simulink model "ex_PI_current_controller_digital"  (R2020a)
settings: Solver=ode45  StartTime=0.0  StopTime=0.1  MaxStep=1e-6  RelTol=1e-4  AbsTol=1e-6  EnableMultiTasking=on
libraries: powerlib x4

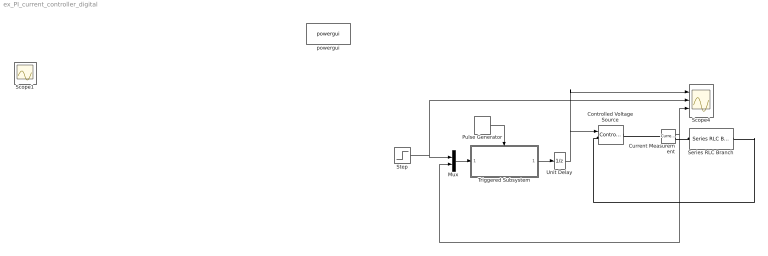
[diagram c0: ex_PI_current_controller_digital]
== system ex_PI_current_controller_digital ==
  Controlled Voltage Source : powerlib/Electrical Sources/Controlled Voltage Source  Initialize=on  Source_Type=AC  Amplitude=0  Phase=0  Frequency=0  Measurements=None
  Current Measurement : powerlib/Measurements/Current Measurement  PhasorSimulation=off  OutputType=Complex  PSBequivalent=0
  Mux : Mux  Inputs=2
  Pulse Generator : DiscretePulseGenerator  PulseType=Time based  Period=0.0001  PulseWidth=50
  Scope4 : Scope  NumInputPorts=3
  Series RLC Branch : powerlib/Elements/Series RLC Branch  LConnTagsString=__new0  RConnTagsString=__new0  BranchType=RL  Resistance=0.1  Inductance=0.001  SetiL0=off  InitialCurrent=0  Capacitance=1e-6  Setx0=off  InitialVoltage=0  Measurements=None
  Step : Step  Time=0.02  After=10  SampleTime=0
  Triggered Subsystem : Subsystem  TreatAsAtomicUnit=on
  Unit Delay : UnitDelay  SampleTime=0.0001  HasFrameUpgradeWarning=on
  powergui : powerlib/powergui  Priority=1  SimulationMode=Continuous  SampleTime=50e-6  frequency=60  Iterations=50  frequencyindice=0  Pbase=100e6  ErrMax=1e-4  UnitsV=kV  UnitsW=MW  buscounter=0  FunctionMessages=off  echomessages=off  EnableUseOfTLC=off  CurrentSourceSwitches=off  DisableSnubberDevices=off  DisableRonSwitches=off  DisableVfSwitches=off  DisplayEquations=off  AutomaticDiscreteSolvers=off  SolverType=Tustin/Backward Euler (TBE)  Interpol=off  ExternalGateDelay=off  methode=off  Ts=100  x0status=blocks  SPID=on  SwTol=0  HookPort=off  NonlinearTolerance=1e-4  nMaxIteration=100  ContinueOnMaxIteration=off  RestoreLinks=warning  ResistiveCurrentMeasurement=off  Frange=[0:2:500]  Ylog=off  Xlog=on  ShowGrid=off  save=off  variable=ZData  structure=0  ZoomFFT=off  StartTime=0.0  cycles=1  DisplayStyle=1  fundamental=60  FreqAxis=off  MaxFrequency=1000  frequencyindicesteady=1  RmsSteady=1  display=off
  Scope1 : Scope
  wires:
  Step/1 -> Mux/1, Scope4/2
  Triggered Subsystem/1(Out1) -> Unit Delay/1
  Current Measurement/1 -> Scope4/3, Mux/2
  Pulse Generator/1 -> Triggered Subsystem/Trigger
  Mux/1 -> Triggered Subsystem/1(In1)
  Unit Delay/1 -> Scope4/1, Controlled Voltage Source/1
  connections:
  Current Measurement/RConn1 -- Series RLC Branch/LConn1
  Controlled Voltage Source/LConn1 -- Series RLC Branch/RConn1
  Controlled Voltage Source/RConn1 -- Current Measurement/LConn1

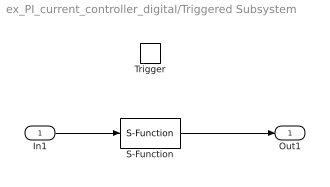
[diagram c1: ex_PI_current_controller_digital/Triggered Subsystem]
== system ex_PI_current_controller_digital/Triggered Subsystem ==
  In1 : Inport
  Trigger : TriggerPort  VariantControl=(inherit)
  S-Function : S-Function  FunctionName=controller  SFunctionDeploymentMode=off  EnableBusSupport=off
  Out1 : Outport
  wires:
  In1/1 -> S-Function/1
  S-Function/1 -> Out1/1
